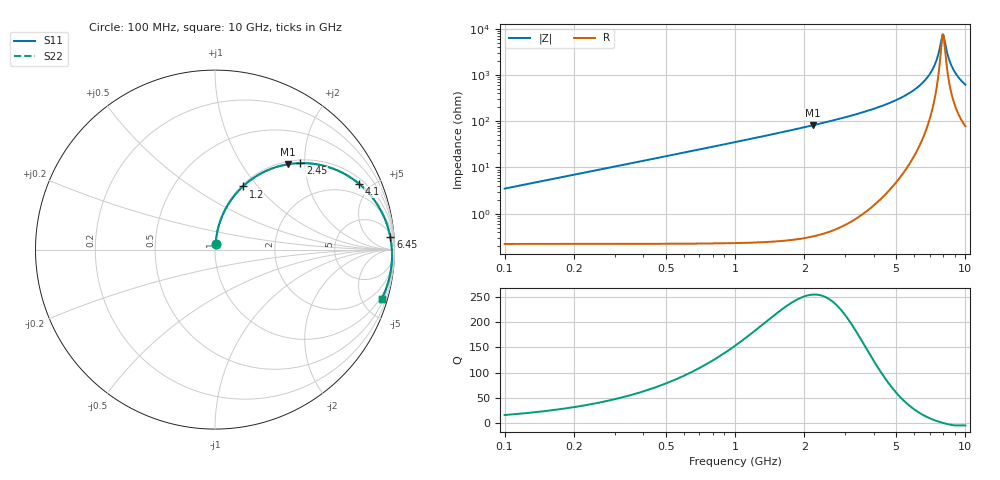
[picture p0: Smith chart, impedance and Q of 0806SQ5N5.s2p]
! Coilcraft 0806SQ-5N5 Air Core Inductor
# MHZ S MA R 50
!Freq  MagS11  AngS11  MagS21  AngS21  MagS12  AngS12  MagS22  AngS22
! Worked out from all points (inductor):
!   397 points, 100 MHz to 10 GHz, reference 50 ohm
!   read as one part in series: L = 5.52 nH near 125 MHz
!   highest Q = 255 at 2.175 GHz (marker M1), where L = 5.96 nH
!   self-resonance near 7.975 GHz
!   S11 on the Smith chart (normalised r, x): 100 MHz: 1.00, +0.07; 1.2 GHz: 1.02, +0.84; 2.45 GHz: 1.07, +1.90; 4.1 GHz: 1.28, +4.23; 6.45 GHz: 8, +26; 10 GHz: 0.75, -6.77
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100  0.03401 84.3  0.9972 -2.0  0.9972 -2.0  0.03401 84.3
225  0.07626 83.8  0.9949 -4.5  0.9949 -4.5  0.07627 83.8
450  0.1515 80.1  0.9863 -9.0  0.9863 -9.0  0.1515 80.1
775  0.2568 74.1  0.9643 -15.4  0.9643 -15.4  0.2568 74.1
1200  0.3849 66.2  0.9208 -23.5  0.9208 -23.5  0.385 66.2
1750  0.5298 56.5  0.8459 -33.3  0.8459 -33.3  0.5298 56.5
2175  0.6239 49.6  0.779 -40.2  0.779 -40.2  0.624 49.6
2450  0.6767 45.4  0.7335 -44.4  0.7335 -44.4  0.6768 45.4
3400  0.8153 32.6  0.5743 -57.1  0.5743 -57.1  0.8154 32.6
4100  0.8824 24.6  0.4627 -64.9  0.4627 -64.9  0.8826 24.6
5050  0.94 15.3  0.325 -73.8  0.325 -73.8  0.9401 15.3
6450  0.9794 4.0  0.153 -82.7  0.153 -82.7  0.9795 4.0
6700  0.9826 2.2  0.126 -83.5  0.126 -83.5  0.9827 2.2
7125  0.986 -0.7  0.08232 -83.3  0.08232 -83.3  0.9862 -0.7
7450  0.9872 -2.7  0.05115 -79.8  0.05115 -79.8  0.9874 -2.7
7650  0.9874 -4.0  0.03328 -72.8  0.03328 -72.8  0.9875 -4.0
7975  0.9869 -5.9  0.01308 -12.9  0.01308 -12.9  0.9871 -5.9
8050  0.9867 -6.4  0.01412 14.4  0.01412 14.4  0.9868 -6.4
8350  0.9853 -8.1  0.03376 57.2  0.03376 57.2  0.9855 -8.1
8625  0.9835 -9.6  0.0553 64.7  0.0553 64.7  0.9837 -9.6
8975  0.9806 -11.5  0.08227 67.3  0.08227 67.3  0.9808 -11.5
10000  0.9687 -16.6  0.1548 66.2  0.1548 66.2  0.9689 -16.6
